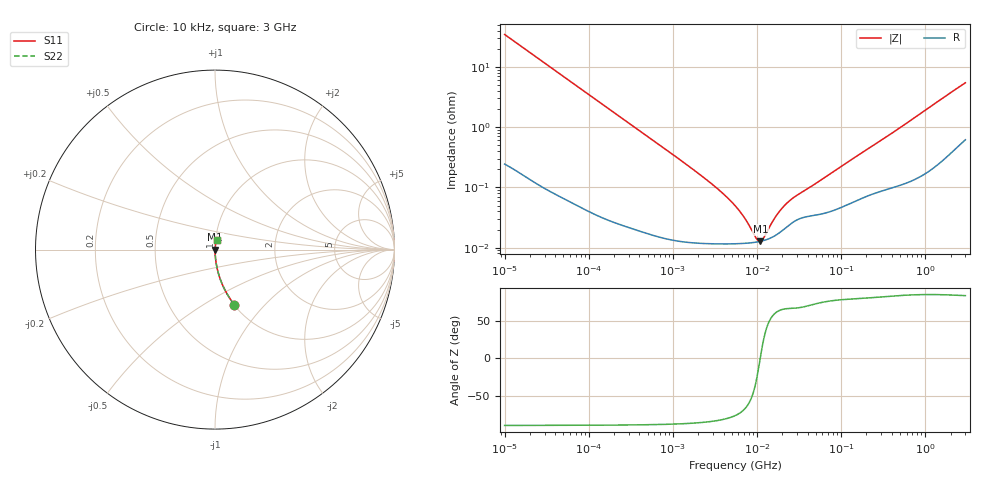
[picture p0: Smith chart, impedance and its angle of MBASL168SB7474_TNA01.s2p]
! MBASL168SB7474_TNA01  S-PARAMETER MODEL  ( Standard Model )
! Model Generated by TAIYO YUDEN Corporation (http://www.ty-top.com)
! Version 1.0
! TAIYO YUDEN Control No. 220601
! Copyright(c) 2012 TAIYO YUDEN CO.,LTD. All Rights Reserved.
! Product Description (link to TY-COMPAS)
! https://ds.yuden.co.jp/TYCOMPAS/or/detail?pn=MBASL168SB7474KTNA01&u=M
! Products Name : Multilayer Ceramic Capacitors
! Characteristics :
!  Capacitance : 0.47 [uF] , Rated Voltage : 10 [V] , TCC : X7R
!  Case Size : 1.6 x 0.8 / 0.063 x 0.031 [mm/inch] , Thickness : 0.8 / 0.031 [mm/inch]
!  (Conditions: Temperature = 25 [degC] , DC Bias Voltage = 0 [V])
! External Node Assignments :
!  1  o---| |---o  2
! GND o---------o GND
! Frequency Range : 10kHz  -  3GHz  [ 401 STEP ]
# MHZ S RI R 50
! Freq[MHz].  S11 Real  S11 Imag  S21 Real  S21 Imag  S12 Real  S12 Imag  S22 Real  S22 Imag
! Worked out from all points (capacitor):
!   401 points, 10 kHz to 3 GHz, reference 50 ohm
!   read as one part in series: C = 462 nF near 10.65 kHz
!   lowest |Z| = 12.7 mohm at 10.96 MHz (marker M1)
!   series resonance near 10.93 MHz, so ESL is about 460 pH
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0.01  0.1077 -0.3065  0.8923 0.3065  0.8923 0.3065  0.1077 -0.3065
0.015549  0.0484 -0.2109  0.9516 0.2109  0.9516 0.2109  0.0484 -0.2109
0.026575  0.0177 -0.1278  0.9823 0.1278  0.9823 0.1278  0.0177 -0.1278
0.045421  0.00648 -0.0758  0.9935 0.0758  0.9935 0.0758  0.00648 -0.0758
0.082683  0.00222 -0.042  0.9978 0.042  0.9978 0.042  0.00222 -0.042
0.199902  0.000567 -0.0175  0.9994 0.0175  0.9994 0.0175  0.000567 -0.0175
0.683653  0.000176 -0.00514  0.9998 0.00514  0.9998 0.00514  0.000176 -0.00514
2.737278  0.000118 -0.00121  0.9999 0.00121  0.9999 0.00121  0.000118 -0.00121
4.124064  0.000116 -0.000738  0.9999 0.000738  0.9999 0.000738  0.000116 -0.000738
5.477226  0.000116 -0.000486  0.9999 0.000486  0.9999 0.000486  0.000116 -0.000486
7.274378  0.000118 -0.000273  0.9999 0.000273  0.9999 0.000273  0.000118 -0.000273
9.6612  0.000123 -8.08e-05  0.9999 8.08e-05  0.9999 8.08e-05  0.000123 -8.08e-05
10.29003  0.000125 -3.93e-05  0.9999 3.93e-05  0.9999 3.93e-05  0.000125 -3.93e-05
10.95979  0.000127 2.04e-06  0.9999 -2.04e-06  0.9999 -2.04e-06  0.000127 2.04e-06
12.04705  0.000132 6.43e-05  0.9999 -6.43e-05  0.9999 -6.43e-05  0.000132 6.43e-05
16.51234  0.000159 0.000279  0.9998 -0.000279  0.9998 -0.000279  0.000159 0.000279
21.24962  0.000206 0.000456  0.9998 -0.000456  0.9998 -0.000456  0.000206 0.000456
27.34599  0.000269 0.000625  0.9997 -0.000625  0.9997 -0.000625  0.000269 0.000625
45.28751  0.00034 0.00101  0.9997 -0.00101  0.9997 -0.00101  0.00034 0.00101
374.4521  0.001 0.00734  0.999 -0.00734  0.999 -0.00734  0.001 0.00734
1991.2  0.00496 0.0366  0.995 -0.0366  0.995 -0.0366  0.00496 0.0366
3000  0.00899 0.0532  0.991 -0.0532  0.991 -0.0532  0.00899 0.0532
